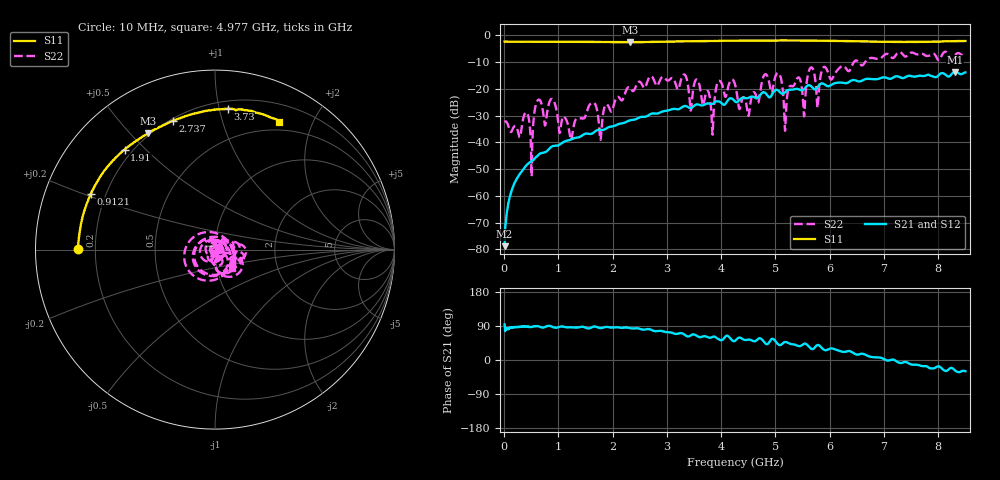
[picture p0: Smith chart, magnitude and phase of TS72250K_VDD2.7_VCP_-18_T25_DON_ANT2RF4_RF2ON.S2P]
!Agilent Technologies,E5071C,MY46417908,A.11.23
!Date: Thu Oct 03 13:33:53 2019
!Data & Calibration Information:
!Freq	S11:SOLT2(ON)	S21:SOLT2(ON)	S12:SOLT2(ON)	S22:SOLT2(ON)
!PortZ  Port1:50+j0  Port2:50+j0
!Above PortZ is port z conversion or system Z0 setting when saving the data.
!When reading, reference impedance value at option line is always used.
# Hz S dB R 50
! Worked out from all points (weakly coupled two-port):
!   1601 points, 10 MHz to 8.5 GHz, reference 50 ohm
!   highest |S21| = -13.67 dB at 8.309 GHz (marker M1); lowest = -78.8 dB at 10 MHz (marker M2)
!   lowest |S11| = -2.5 dB at 2.329 GHz (marker M3), VSWR 6.90, Z = 9.59 + j28.1 ohm
!   |S11| at or under -10 dB: nowhere
!   |S22| runs from -52.7 to -6.1 dB; largest |S21 - S12| = 0.0017
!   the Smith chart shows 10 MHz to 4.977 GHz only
!   S11 on the Smith chart (normalised r, x): 10 MHz: 0.13, +0.00; 912.1 MHz: 0.14, +0.21; 1.91 GHz: 0.17, +0.43; 2.737 GHz: 0.21, +0.71; 3.73 GHz: 0.26, +1.06; 4.977 GHz: 0.39, +1.55
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1e7  -2.32 179.8  -78.76 93.6  -78.65 83.4  -32.38 1.5
2.275562e8  -2.38 173.5  -53.83 86.6  -53.80 87.5  -34.32 2.0
9.120625e8  -2.40 155.8  -41.30 86.1  -41.31 85.7  -24.34 -37.0
1.230438e9  -2.41 148.1  -38.89 86.5  -38.92 86.3  -38.98 -89.6
1.426769e9  -2.43 143.6  -37.56 87.9  -37.59 87.6  -30.94 90.2
1.909638e9  -2.49 132.1  -34.47 87.1  -34.44 87.0  -26.06 56.5
2.328831e9  -2.53 120.0  -31.70 83.8  -31.66 83.7  -19.81 13.0
2.737412e9  -2.44 108.0  -29.17 78.0  -29.13 77.8  -15.73 -15.9
2.843538e9  -2.41 105.0  -29.13 76.8  -29.08 76.9  -18.18 -6.5
3.729681e9  -2.07 84.9  -25.52 61.7  -25.52 61.9  -21.07 -65.6
3.835806e9  -2.05 82.8  -25.63 60.5  -25.64 60.7  -35.72 -94.6
3.952544e9  -2.06 81.2  -24.68 55.1  -24.69 55.2  -17.05 -88.9
4.255e9  -1.96 75.7  -24.68 50.6  -24.67 50.6  -18.32 -173.4
4.499088e9  -1.96 71.6  -23.39 53.8  -23.38 53.8  -30.06 -128.3
4.97665e9  -1.95 63.3  -20.86 53.5  -20.83 53.8  -17.11 -47.0
5.183594e9  -1.92 59.6  -21.10 47.6  -21.09 47.8  -33.39 -114.3
5.671769e9  -1.93 51.9  -19.29 29.0  -19.29 29.3  -12.02 -166.7
5.777894e9  -1.99 50.4  -19.32 39.6  -19.36 40.0  -27.11 -154.2
5.894631e9  -1.99 48.5  -18.20 27.1  -18.22 27.3  -11.79 -158.1
7.088538e9  -2.40 25.1  -16.15 -1.4  -16.19 -1.4  -7.20 158.8
8.308975e9  -2.14 -0.8  -13.67 -27.5  -13.68 -27.4  -7.47 130.0
8.5e9  -2.11 -2.9  -13.82 -29.6  -13.87 -29.9  -7.56 113.7
